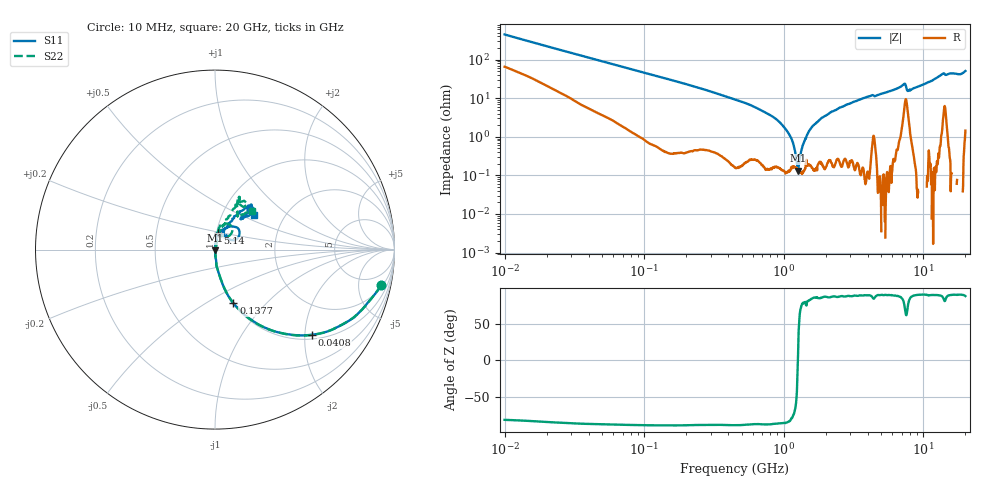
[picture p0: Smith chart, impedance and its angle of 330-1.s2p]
!Keysight Technologies,P5008B,MY61100088,A.16.20.02
!Date: Monday, May 27, 2024 17:43:22
!Correction: S11(C* 2-Port  )
!S21(C* 2-Port  )
!S12(C* 2-Port  )
!S22(C* 2-Port  )
!S2P File: Measurements: S11, S21, S12, S22:Log Frequency Sweep
# Hz S  dB  R 50
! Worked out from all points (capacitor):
!   1601 points, 10 MHz to 20 GHz, reference 50 ohm
!   read as one part in series: C = 36.2 pF near 10.39 MHz
!   lowest |Z| = 131 mohm at 1.266 GHz (marker M1)
!   series resonance near 1.262 GHz, so ESL is about 440 pH
!   S11 on the Smith chart (normalised r, x): 10 MHz: 2.22, -8.85; 40.8 MHz: 1.11, -2.18; 137.7 MHz: 1.01, -0.67; 5.14 GHz: 1.01, +0.19; 20 GHz: 1.40, +0.59
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1e7  -0.46 -12.1  -13.45 69.5  -13.46 69.5  -0.48 -12.1
3.555162e7  -2.38 -37.5  -4.29 49.4  -4.30 49.4  -2.38 -37.5
4.080285e7  -2.86 -41.3  -3.60 46.0  -3.61 46.0  -2.86 -41.4
1.263918e8  -9.37 -69.5  -0.58 19.8  -0.59 19.8  -9.36 -69.5
1.376751e8  -10.01 -71.1  -0.50 18.4  -0.51 18.4  -10.00 -71.0
4.472136e8  -20.54 -84.4  -0.05 5.1  -0.06 5.1  -20.54 -84.2
9.119826e8  -30.32 -86.2  -0.01 1.2  -0.02 1.2  -30.41 -84.9
1.145559e9  -37.39 -84.3  -0.00 0.1  -0.02 0.2  -37.20 -78.1
1.265737e9  -46.25 -82.8  -0.00 -0.3  -0.01 -0.3  -44.32 -61.9
1.339989e9  -57.91 -93.8  -0.00 -0.6  -0.01 -0.6  -49.21 -30.6
1.385298e9  -65.65 68.9  -0.00 -0.7  -0.01 -0.7  -49.35 1.1
1.480564e9  -45.32 72.3  -0.00 -1.1  -0.01 -1.1  -43.88 44.8
1.589917e9  -38.85 85.2  -0.00 -1.4  -0.01 -1.4  -39.10 66.3
1.88646e9  -32.54 84.9  0.00 -2.3  -0.01 -2.3  -32.87 73.1
2.496738e9  -27.15 82.5  -0.00 -3.9  -0.01 -3.9  -27.32 76.9
5.140092e9  -20.70 81.2  -0.02 -9.9  -0.03 -9.9  -20.64 76.1
5.652411e9  -19.73 76.9  -0.03 -11.1  -0.04 -11.1  -19.76 79.1
7.236311e9  -15.54 49.5  -0.41 -16.1  -0.42 -16.1  -16.04 68.2
7.995456e9  -19.78 51.6  -0.13 -13.6  -0.14 -13.7  -20.51 77.7
1.018741e10  -18.35 65.4  -0.02 -19.9  -0.03 -19.9  -18.41 73.3
1.367661e10  -10.36 51.0  -0.49 -29.3  -0.50 -29.3  -10.36 61.8
2e10  -10.76 41.9  -0.44 -41.9  -0.45 -41.9  -10.53 46.8
